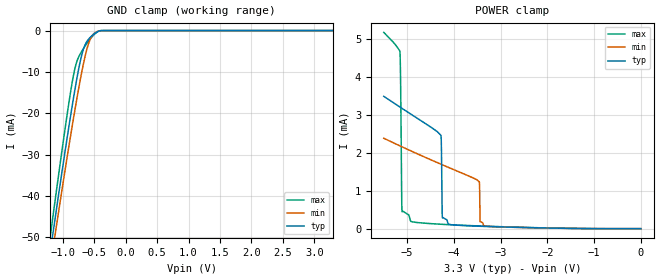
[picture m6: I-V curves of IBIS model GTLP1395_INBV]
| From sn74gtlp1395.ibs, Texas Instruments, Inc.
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[Model]   GTLP1395_INBV
Model_type  Input
Vinl = 0.8
Vinh = 2.0
| variable   typ   min   max
C_comp   3.36pF   2.44pF   5.01pF
[Temperature Range]   40   100   -40
| Ambient temperature   25   85   -40
[Voltage range]   3.3   3.15   3.45
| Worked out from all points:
|   GND clamp passes 1 mA (typ) near -0.52 V on its own axis
|   POWER clamp passes 1 mA (typ) near -4.26 V on its own axis
[GND Clamp]
| GTLP1395_INBV_
|   Voltage   I(typ)   I(min)   I(max)
-5.5V     -543.7mA   -522.7mA   -576.6mA
-1.225V   -56.2mA    -59.65mA   -52.62mA
-1.18V    -51.43mA   -55.09mA   -47.52mA
-1.14V    -47.22mA   -51.06mA   -43mA
-1.1V     -43.05mA   -47.06mA   -38.52mA
-920mV    -24.81mA   -29.52mA   -19.1mA
-810mV    -14.46mA   -19.37mA   -9.307mA
-730mV    -7.943mA   -12.5mA    -5.842mA
-665mV    -4.167mA   -7.527mA   -4.182mA
-580mV    -1.886mA   -2.683mA   -2.327mA
-485mV    -598uA     -480.8uA   -727.2uA
3.3V      223.5pA    719pA      1.745nA
[POWER Clamp]
| GTLP1395_INBV
|   Voltage   I(typ)   I(min)   I(max)
-5.5V     3.491mA    2.385mA    5.177mA
-5.155V   3.209mA    2.185mA    4.682mA
-5.14V    3.197mA    2.176mA    3.899mA
-5.11V    3.173mA    2.159mA    448.3uA
-4.92V    3.02mA     2.051mA    192.8uA
-4.275V   2.454mA    1.7mA      116.3uA
-4.245V   281.5uA    1.684mA    114.3uA
-4.115V   121.8uA    1.615mA    105.9uA
-3.455V   63.49uA    1.232mA    71.72uA
-3.44V    62.83uA    185.2uA    71.06uA
-3.345V   58.83uA    74.81uA    66.93uA
-95.1fV   223.5pA    707.2pA    1.774nA
